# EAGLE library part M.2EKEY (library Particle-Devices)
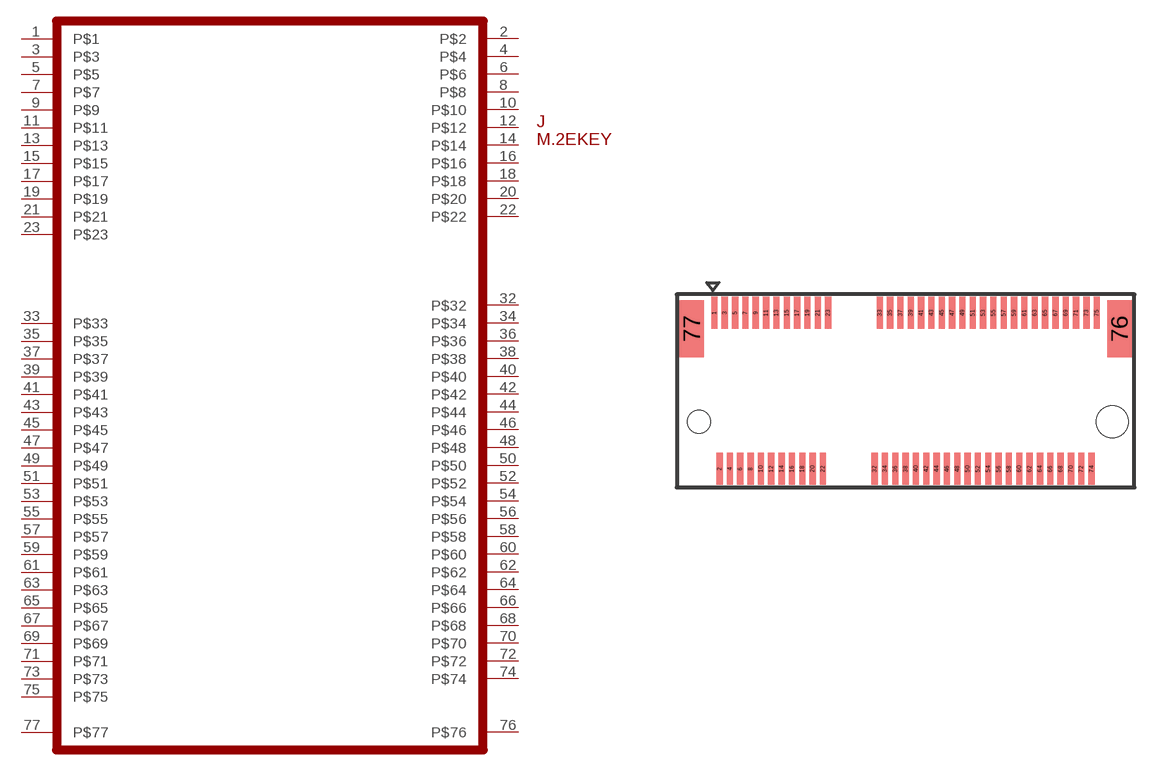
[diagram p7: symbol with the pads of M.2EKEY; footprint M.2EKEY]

Designator prefix J

## M.2EKEY  [M.2EKEY]
1  P$1
2  P$2
3  P$3
4  P$4
5  P$5
6  P$6
7  P$7
8  P$8
9  P$9
10  P$10
11  P$11
12  P$12
13  P$13
14  P$14
15  P$15
16  P$16
17  P$17
18  P$18
19  P$19
20  P$20
21  P$21
22  P$22
23  P$23
32  P$32
33  P$33
34  P$34
35  P$35
36  P$36
37  P$37
38  P$38
39  P$39
40  P$40
41  P$41
42  P$42
43  P$43
44  P$44
45  P$45
46  P$46
47  P$47
48  P$48
49  P$49
50  P$50
51  P$51
52  P$52
53  P$53
54  P$54
55  P$55
56  P$56
57  P$57
58  P$58
59  P$59
60  P$60
61  P$61
62  P$62
63  P$63
64  P$64
65  P$65
66  P$66
67  P$67
68  P$68
69  P$69
70  P$70
71  P$71
72  P$72
73  P$73
74  P$74
75  P$75
76  P$76  pwr
77  P$77  pwr

## Footprint M.2EKEY (pad centres in mm)
smd 0.3 x 1.55: 1 -9.62,3.735; 2 -9.37,-3.815; 3 -9.12,3.735; 4 -8.87,-3.815; 5 -8.62,3.735; 6 -8.37,-3.815; 7 -8.12,3.735; 8 -7.87,-3.815; 9 -7.62,3.735; 10 -7.37,-3.815; 11 -7.12,3.735; 12 -6.87,-3.815; 13 -6.62,3.735; 14 -6.37,-3.815; 15 -6.12,3.735; 16 -5.87,-3.815; 17 -5.62,3.735; 18 -5.37,-3.815; 19 -5.12,3.735; 20 -4.87,-3.815; 21 -4.62,3.735; 22 -4.37,-3.815; 23 -4.12,3.735; 32 -1.87,-3.815; 33 -1.62,3.735; 34 -1.37,-3.815; 35 -1.12,3.735; 36 -0.87,-3.815; 37 -0.62,3.735; 38 -0.37,-3.815; 39 -0.12,3.735; 40 0.13,-3.815; 41 0.38,3.735; 42 0.63,-3.815; 43 0.88,3.735; 44 1.13,-3.815; 45 1.38,3.735; 46 1.63,-3.815; 47 1.88,3.735; 48 2.13,-3.815; 49 2.38,3.735; 50 2.63,-3.815; 51 2.88,3.735; 52 3.13,-3.815; 53 3.38,3.735; 54 3.63,-3.815; 55 3.88,3.735; 56 4.13,-3.815; 57 4.38,3.735; 58 4.63,-3.815; 59 4.88,3.735; 60 5.13,-3.815; 61 5.38,3.735; 62 5.63,-3.815; 63 5.88,3.735; 64 6.13,-3.815; 65 6.38,3.735; 66 6.63,-3.815; 67 6.88,3.735; 68 7.13,-3.815; 69 7.38,3.735; 70 7.63,-3.815; 71 7.88,3.735; 72 8.13,-3.815; 73 8.38,3.735; 74 8.63,-3.815; 75 8.88,3.735
smd 1.2 x 2.75: 76 9.98,2.96; 77 -10.72,2.96
hole 1.1 at -10.37,-1.54
hole 1.55 at 9.63,-1.54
